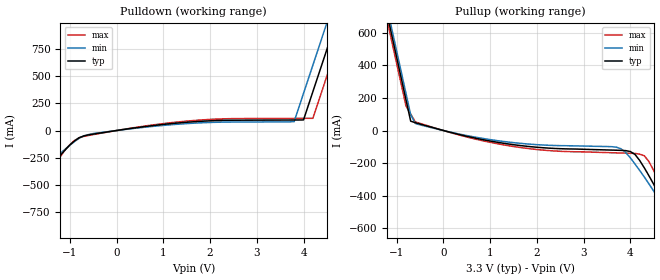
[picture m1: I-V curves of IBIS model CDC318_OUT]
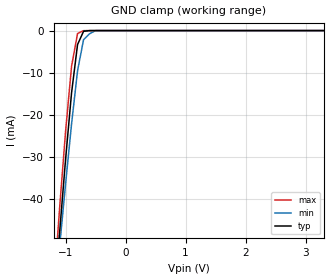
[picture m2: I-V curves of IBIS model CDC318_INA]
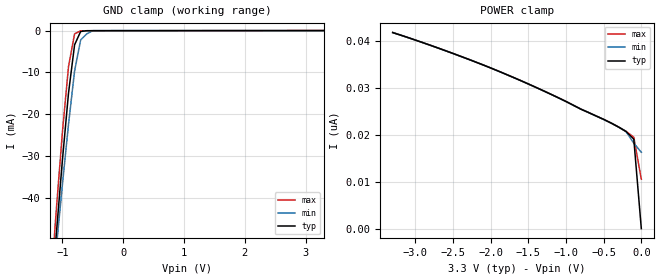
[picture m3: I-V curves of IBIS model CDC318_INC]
[IBIS Ver]   2.1
[File Name]   cd318e21.ibs  | This IBIS file is for DEVICE: CDC318ADL
[File Rev]   2.1
[Date]   10/22/98
[Source]   file originated at Texas Instruments
[Notes]   The following information corresponds to the
|   CDC318E-DIE output buffers and input ESD circuits.
|Revision log: 2.0, 03/19/98 IBIS model for the CDC318D1 chip. It uses the same
|   output plots as for CDC318D, but the internal slew
|   rate has been ajusted to according to D1 characte-
|   ristics.
|   Since the production version of D1 chip will be
|   called CDC318E, the module name was set to the
|   production chip revision "E" instead of "D1".
|   2.1, 10/22/98 Put device name behind the file name
[Disclaimer] This information is for modeling purposes only
|and is not guaranteed.
|Property of Texas Instruments Incorporated unauthorized reproduction
|and/or distribution is strictly prohibited.
|This product is protected under copyright law and trade
|secret law as an unpublished work.  Created  1997.
|(C) Copyright 1997 Texas Instruments Incorporated.
|All rights reserved.
|These commodities are under U.S. Government distribution
|license control. As such, they are not to be re-exported
|without prior approval of the U.S. Department of Commerce.
|Please be aware that in the absence of a written agreement
|to the contrary, Texas Instruments ("TI") assumes no
|liability for:  (1) the accuracy of the IBIS Models provided
|to your company;  (2) the proper functioning of these Models
|in your design system or for any resulting applications;
|or (3) infringement of patents, copyrights or intellectual
|property rights resulting from your use of these models.
|TI provides IBIS Models as a service to our customers
|and therefore reserves the right to limit distribution
|of the Models.
|CDC318 IBIS I/O Model
|Mixed Signal Products, Texas Instruments
[Component]   CDC318E-DIE
[Manufacturer] Texas Instruments
[Package]
|   typ   min   max
R_pkg   0.036   0.026   0.041
L_pkg   5.63n   4.598n   7.833n
C_pkg   0.76p   0.407p   1.120p
[Pin]   signal_name   model_name   R_pin   L_pin   C_pin
1   NC   NC   0.041   7.83n   0.97p
2   NC   NC   0.041   7.19n   1.12p
3   VCC   POWER   0.041   6.69n   1.03p
4   1Y0   CDC318_OUT   0.041   6.24n   0.91p
5   1Y1   CDC318_OUT   0.035   5.79n   0.85p
6   GND   GND   0.026   5.33n   0.82p
7   VCC   POWER   0.035   5.02n   0.76p
8   1Y2   CDC318_OUT   0.035   4.87n   0.63p
9   1Y3   CDC318_OUT   0.036   4.75n   0.55p
10   GND   GND   0.036   4.65n   0.54p
11   A   CDC318_INA   0.035   4.60n   0.53p
12   VCC   POWER   0.036   4.61n   0.41p
13   2Y0   CDC318_OUT   0.036   4.61n   0.41p
14   2Y1   CDC318_OUT   0.035   4.60n   0.53p
15   GND   GND   0.036   4.65n   0.54p
16   VCC   POWER   0.036   4.75n   0.55p
17   2Y2   CDC318_OUT   0.035   4.87n   0.63p
18   2Y3   CDC318_OUT   0.035   5.02n   0.76p
19   GND   GND   0.026   5.33n   0.82p
20   VCC   POWER   0.035   5.79n   0.85p
21   5Y0   CDC318_OUT   0.041   6.24n   0.91p
22   GND   GND   0.041   6.69n   1.03p
23   VCC   POWER   0.041   7.19n   1.12p
24   SDATA   CDC318_IO   0.041   7.83n   0.97p
25   SCLOCK   CDC318_INC   0.041   7.83n   0.97p
26   GND   GND   0.041   7.19n   1.12p
27   GND   GND   0.041   6.69n   1.03p
28   5Y1   CDC318_OUT   0.041   6.24n   0.91p
29   VCC   POWER   0.035   5.79n   0.85p
30   GND   GND   0.026   5.33n   0.82p
31   3Y0   CDC318_OUT   0.035   5.02n   0.76p
32   3Y1   CDC318_OUT   0.035   4.87n   0.63p
33   VCC   POWER   0.036   4.75n   0.55p
34   GND   GND   0.036   4.65n   0.54p
35   3Y2   CDC318_OUT   0.035   4.60n   0.53p
36   3Y3   CDC318_OUT   0.036   4.61n   0.41p
37   VCC   POWER   0.036   4.61n   0.41p
38   OE   CDC318_INE   0.035   4.60n   0.53p
39   GND   GND   0.036   4.65n   0.54p
40   4Y0   CDC318_OUT   0.036   4.75n   0.55p
41   4Y1   CDC318_OUT   0.035   4.87n   0.63p
42   VCC   POWER   0.035   5.02n   0.76p
43   GND   GND   0.026   5.33n   0.82p
44   4Y2   CDC318_OUT   0.035   5.79n   0.85p
45   4Y3   CDC318_OUT   0.041   6.24n   0.91p
46   VCC   POWER   0.041   6.69n   1.03p
47   NC   NC   0.041   7.19n   1.12p
48   NC   NC   0.041   7.83n   0.97p
| Models and submodels in the file (5): CDC318_OUT (3-state), CDC318_INA (Input), CDC318_INC (Input), CDC318_INE (Input), CDC318_IO (I/O_open_drain)
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|   Model CDC318_OUT
[Model]   CDC318_OUT
Model_type   3-state
Polarity   Non-Inverting
Enable   Active-High
Vmeas = 1.5V
Cref = 30pF
Rref = 500
Vref = 0
|   variable   typ   min   max
C_comp   5.2pF   NA   NA
[Voltage range]   3.3   3.135   3.465
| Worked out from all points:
|   slope of the pulldown table from 0 to 0.495 V, typ, clamps not added: 16.3 ohm
|   slope of the pullup table from 0 to 0.495 V, typ, clamps not added: 14 ohm
[Pullup]
| Voltage   I(typ)   I(min)   I(max)
-3.3V     3.449A     3.489A     3.408A
-1.2V     709.6mA    748.9mA    671.5mA
-1.1V     579.1mA    618.4mA    541.2mA
-800mV    187.8mA    227mA      150.2mA
-700mV    57.37mA    96.46mA    101.5mA
-500mV    39.83mA    34.89mA    43.83mA
1.2V      -74.3mA    -63.93mA   -83.57mA
3.7V      -121mA     -102.4mA   -137.2mA
4V        -129.1mA   -168mA     -139.8mA
4.4V      -279.4mA   -328.7mA   -192.2mA
5.1V      -655.3mA   -638mA     -632.1mA
6.6V      -1.478A    -1.309A    -1.641A
[Pulldown]
|  Voltage   I(typ)   I(min)   I(max)
-3.3V     -1.358A    -1.089A    -1.673A
-2.6V     -977.5mA   -792.4mA   -1.195A
-2.2V     -761.1mA   -623.8mA   -923.2mA
-1.2V     -228.2mA   -209.6mA   -238.8mA
-800mV    -66.4mA    -71.48mA   -66.52mA
3.8V      97.08mA    82.28mA    112.3mA
4V        97.84mA    342.8mA    112.6mA
4.2V      358.2mA    603.3mA    112.9mA
4.5V      748.7mA    994mA      503mA
4.7V      1.009A     1.255A     763mA
4.9V      1.269A     1.515A     1.023A
6.6V      3.482A     3.729A     3.233A
[Ramp]
|  variable   typ   min   max
dV/dt_r   2.00/1.40n   2.00/1.70n   2.00/1.00n
dV/dt_f   2.00/1.30n   2.00/1.60n   2.00/0.90n
|   Model CDC318_INA
[Model]   CDC318_INA
Model_type   Input
Polarity   Non-Inverting
Vinl = 0.8V
Vinh = 2.0V
Vmeas = 1.5V
| variable   typ   min   max
C_comp   3.2p   NA   NA
[Voltage range]   3.3   3.135   3.465
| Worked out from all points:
|   GND clamp passes 1 mA (typ) near -0.73 V on its own axis
[GND_Clamp]
|  Voltage   I(typ)   I(min)   I(max)
-3.3V     -477.3mA   -422.8mA   -533mA
-1.2V     -66.54mA   -66.75mA   -62.4mA
-1.1V     -48.28mA   -51.62mA   -42.53mA
-1V       -30.77mA   -36.6mA    -24.1mA
-900mV    -14.85mA   -22.28mA   -8.521mA
-800mV    -3.326mA   -9.56mA    -712.5uA
-700mV    -173.3uA   -2.174mA   -14.74uA
-600mV    -5.362uA   -765uA     -265.9nA
-500mV    -161.3nA   -3.461uA   -4.802nA
3.3V      106.3pA    107.3pA    106.1pA
|   Model CDC318_INC
[Model]   CDC318_INC
Model_type   Input
Polarity   Non-Inverting
Vinl = 0.99V
Vinh = 2.31V
Vmeas = 1.5V
| variable   typ   min   max
C_comp   3.2p   NA   NA
[Voltage range]   3.3   3.135   3.465
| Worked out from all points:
|   GND clamp passes 1 mA (typ) near -0.72 V on its own axis
[GND_Clamp]
|  Voltage   I(typ)   I(min)   I(max)
-3.3V     -478mA     -423.4mA   -533.7mA
-1.2V     -66.69mA   -66.89mA   -62.55mA
-1.1V     -48.41mA   -51.75mA   -42.66mA
-1V       -30.87mA   -36.7mA    -24.21mA
-900mV    -14.93mA   -22.37mA   -8.601mA
-800mV    -3.388mA   -9.625mA   -775.4uA
-700mV    -218.1uA   -2.221mA   -61.94uA
-600mV    -36.36uA   -795.8uA   -39.76uA
-500mV    -26.09uA   -21.32uA   -38.08uA
3.3V      -9.608pA   30.25nA    -792.1nA
[POWER_clamp]
|  Voltage   I(typ)   I(min)   I(max)
-3.3V     41.72nA    41.71nA    41.76nA
-2.5V     37.28nA    37.27nA    37.29nA
-1.7V     32.19nA    32.18nA    32.2nA
-1.2V     28.6nA     28.59nA    28.61nA
-800mV    25.41nA    25.44nA    25.42nA
-500mV    23.26nA    23.24nA    23.25nA
-200mV    20.65nA    20.61nA    20.69nA
-100mV    19.07nA    18.18nA    19.45nA
0V        9.608pA    16.26nA    10.53nA
